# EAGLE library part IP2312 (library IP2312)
ESOP-8L DC-DC Converters RoHS Source: Datasheet
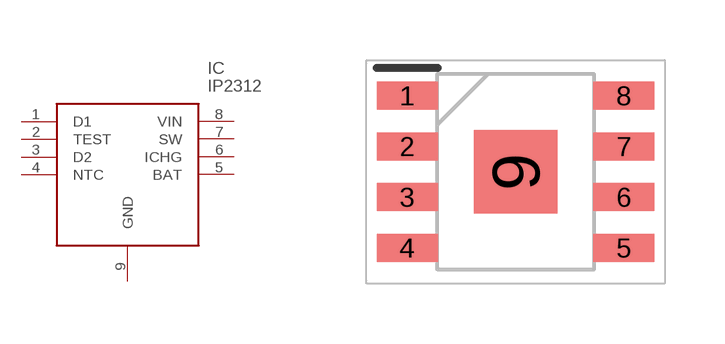
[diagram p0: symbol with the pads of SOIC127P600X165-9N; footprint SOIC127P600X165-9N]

Designator prefix IC

## IP2312 (Description: ESOP-8L DC-DC Converters RoHS; Height: 1.65mm; Manufacturer_Name: INJOINIC; Manufacturer_Part_Number: IP2312)  [SOIC127P600X165-9N]
1  D1
2  TEST
3  D2
4  NTC
5  BAT
6  ICHG
7  SW
8  VIN
9  GND

## Footprint SOIC127P600X165-9N (pad centres in mm)
ESOP-8
smd 1.525 x 0.7: 1 -2.712,1.905; 2 -2.712,0.635; 3 -2.712,-0.635; 4 -2.712,-1.905; 5 2.712,-1.905; 6 2.712,-0.635; 7 2.712,0.635; 8 2.712,1.905
smd 2.09 x 2.09: 9 0,0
